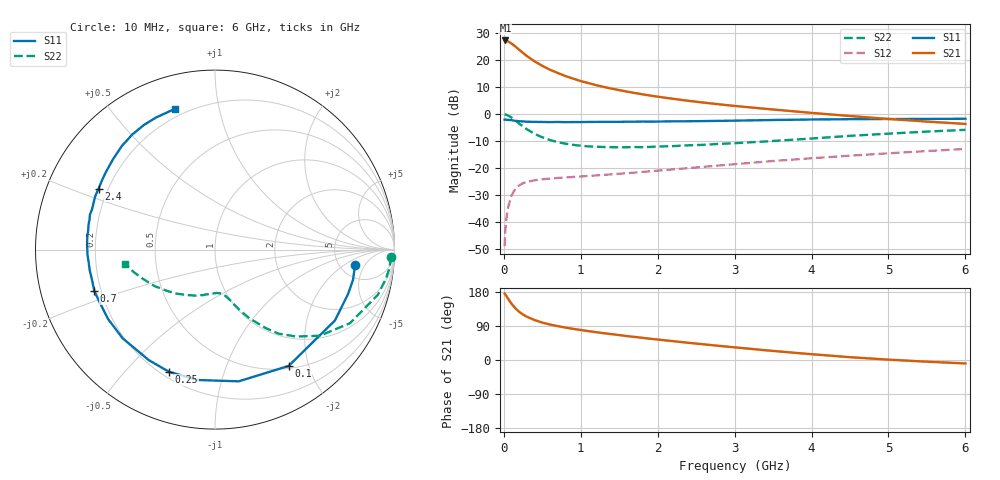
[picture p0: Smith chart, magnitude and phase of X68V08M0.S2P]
! SIEMENS Small Signal Semiconductors
! BFP193W
! Si NPN RF Bipolar Junction Transistor in SOT343
! VCE = 8 V  IC = 8 mA
! Common Emitter S-Parameters:  April 1994
# GHz  S  MA  R  50
!  f  S11  S21  S12  S22
! GHz  MAG  ANG  MAG  ANG  MAG  ANG  MAG  ANG
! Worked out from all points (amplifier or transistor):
!   40 points, 10 MHz to 6 GHz, reference 50 ohm
!   highest |S21| = 27.2 dB at 20 MHz (marker M1)
!   |S21| within 3 dB of that: start of sweep to 181.3 MHz
!   unconditionally stable (mu >= 1): 1.477 GHz to 4.383 GHz
!   at 200 MHz: K = 0.19, MSG = 25.1 dB, |S12| = -26.4 dB
!   at 1.5 GHz: K = 1.01, MAG = 14.8 dB, |S12| = -22.1 dB
!   at 6 GHz: K = 0.92, MSG = 4.6 dB, |S12| = -12.9 dB
!   lowest NFmin = 1.25 dB at 450 MHz
!   S11 on the Smith chart (normalised r, x): 10 MHz: 6.97, -3.04; 100 MHz: 0.54, -1.69; 250 MHz: 0.23, -0.67; 700 MHz: 0.17, -0.16; 2.4 GHz: 0.16, +0.24; 6 GHz: 0.16, +0.74
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0.01  0.7853 -6.1  22.75 175.5  0.0036 88.0  0.9836 -2.4
0.02  0.7872 -12.4  22.8 173.0  0.0072 84.5  0.9757 -6.5
0.05  0.7762 -30.6  22.07 163.2  0.0176 74.8  0.9417 -15.5
0.1  0.7671 -57.7  20.02 148.5  0.0312 62.9  0.8566 -28.6
0.15  0.7457 -79.8  17.63 136.4  0.0414 52.9  0.7562 -39.4
0.2  0.7327 -97.4  15.31 127.0  0.0478 46.0  0.6622 -47.0
0.25  0.7275 -110.6  13.4 119.9  0.0527 40.9  0.5857 -53.0
0.3  0.7177 -120.9  11.73 114.1  0.0555 37.2  0.5195 -57.2
0.4  0.7135 -136.2  9.361 105.3  0.0595 32.3  0.4292 -63.3
0.5  0.7102 -147.0  7.742 98.7  0.0622 30.4  0.3701 -67.4
0.6  0.7065 -155.1  6.555 93.6  0.0637 29.2  0.3294 -70.4
0.7  0.7109 -161.1  5.719 89.4  0.0656 29.0  0.3011 -72.6
0.9  0.7075 -170.5  4.492 82.2  0.0684 29.5  0.2682 -76.7
1.1  0.711 -177.7  3.713 76.2  0.0715 30.8  0.251 -80.3
1.3  0.714 176.3  3.152 70.7  0.0748 32.7  0.2449 -84.0
1.6  0.7183 168.7  2.588 63.1  0.0805 35.6  0.2425 -89.3
2.2  0.7306 156.1  1.905 49.7  0.0944 39.9  0.2544 -101.3
2.4  0.7323 152.3  1.747 45.4  0.0997 40.9  0.2632 -105.1
3.2  0.7597 138.2  1.321 29.6  0.1243 42.9  0.299 -122.0
4.5  0.7994 119.7  0.915 7.4  0.1692 40.4  0.3934 -148.9
5.5  0.8084 110.2  0.722 -4.4  0.2059 36.4  0.4715 -164.8
6  0.8156 105.8  0.654 -9.1  0.2256 34.2  0.508 -171.2
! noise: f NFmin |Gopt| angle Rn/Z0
0.45  1.25  0.23  133  0.12
0.9  1.3  0.35  156  0.11
1.8  2  0.55  -155  0.13
